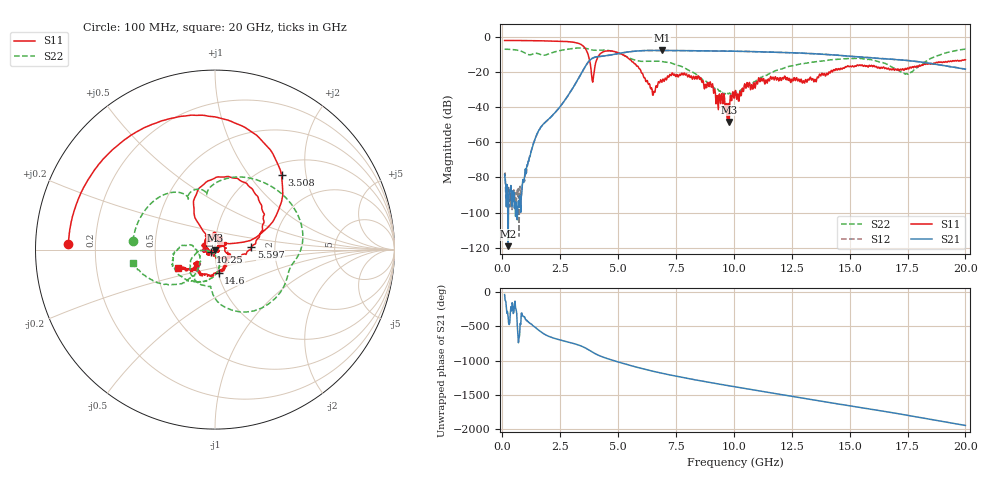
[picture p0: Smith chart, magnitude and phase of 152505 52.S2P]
!  2-Port S-parameters saved by WinCal
! VAR MeasName=S-Parameters (CALIBRATED_DATA) read from VNA (N5230C)
! VAR MeasDate=4/10/2015 9:33:49 AM
! VAR NAME=152505 52
! VAR FILENAME=152505 52.S2P
! VAR DATE=4/10/2015 9:33:49 AM
! VAR PHYS_PORTS=1,2
# Hz S DB R 50
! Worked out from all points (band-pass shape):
!   801 points, 100 MHz to 20 GHz, reference 50 ohm
!   highest |S21| = -7.42 dB at 6.891 GHz (marker M1); lowest = -119.2 dB at 249.2 MHz (marker M2)
!   |S21| within 3 dB of the highest: 4.499 GHz to 14.68 GHz (10.18 GHz wide, 106 % of centre)
!   lowest |S11| = -48.3 dB at 9.801 GHz (marker M3), VSWR 1.01, Z = 49.9 - j0.377 ohm
!   |S11| at or under -10 dB: 3.71 GHz to 4.19 GHz (480.5 MHz wide, 12.2 % of centre); 5.215 GHz to end of sweep
!   |S22| runs from -32.6 to -6.0 dB; largest |S21 - S12| = 0.0057
!   S11 on the Smith chart (normalised r, x): 100 MHz: 0.10, +0.02; 3.508 GHz: 1.22, +1.46; 5.597 GHz: 1.51, +0.05; 10.25 GHz: 0.95, -0.02; 14.6 GHz: 1.01, -0.26; 20 GHz: 0.65, -0.14
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1e8  -1.75 177.6  -78.27 -38.6  -78.72 -85.2  -6.75 173.9
2.4925e8  -1.75 174.1  -119.22 4.6  -95.48 7.7  -6.80 164.6
9.4575e8  -1.82 157.3  -81.12 0.1  -81.60 -7.6  -8.66 121.1
1.5925e9  -1.92 140.9  -52.69 156.6  -52.91 156.3  -9.48 101.0
3.43325e9  -4.32 56.5  -20.03 -72.6  -20.07 -72.6  -6.02 15.7
3.507875e9  -5.10 48.1  -18.30 -83.8  -18.33 -83.9  -6.07 10.4
3.905875e9  -25.57 75.6  -11.79 -160.4  -11.82 -160.5  -7.25 -11.9
4.42825e9  -7.90 89.1  -10.57 120.3  -10.62 119.9  -7.28 -37.4
5.597375e9  -13.81 4.3  -7.99 1.3  -8.02 1.2  -12.39 -93.4
6.492875e9  -32.96 -109.9  -7.45 -75.9  -7.47 -75.6  -13.61 -106.5
6.741625e9  -25.30 167.9  -7.44 -94.6  -7.44 -94.9  -13.55 -116.1
6.890875e9  -25.63 156.5  -7.42 -105.7  -7.46 -105.7  -13.80 -121.3
8.482875e9  -22.20 67.8  -7.67 148.8  -7.63 149.0  -22.28 -176.4
9.80125e9  -48.33 -100.2  -7.84 70.6  -7.82 70.7  -31.76 -123.4
1.005e10  -30.96 -126.6  -7.89 55.9  -7.91 55.8  -32.28 -97.6
1.0249e10  -31.59 -155.0  -7.95 44.7  -7.94 44.7  -30.50 -91.9
1.116938e10  -23.48 -179.5  -8.24 -7.4  -8.20 -7.5  -22.79 -68.8
1.338325e10  -23.83 22.1  -9.29 -130.9  -9.27 -130.6  -14.08 -113.7
1.460212e10  -17.75 -81.3  -10.36 161.4  -10.29 161.1  -12.39 -141.6
1.669162e10  -17.86 -141.1  -12.37 47.9  -12.35 47.2  -15.96 171.4
1.75125e10  -17.47 -135.1  -13.26 0.5  -13.23 0.4  -21.01 -156.9
2e10  -12.81 -153.7  -18.13 -146.7  -18.13 -146.2  -6.65 -170.4
